|   IBIS model for TI xxx DSP
[IBIS Ver]   5.1
[Disclaimer]   Please be aware that in the absence of a written agreement
|   Texas Instruments(TI) assumes no liability for:
|   (1) The accuracy of the IBIS models provided to your company,
|   however, the IBIS model is compliant to industry standard
|   IQ Level 2a.  Refer to IBIS Quality Section below for
|   for full details.
|   (2) The proper functioning of these Models in your design
|   or for any resulting applications
|   (3) Infringement of patents, copyrights or intellectual
|   property rights resulting from your use of these
|   models.
|   TI provides IBIS Models as a service to our customers and
|   therefore reserves the right to limit distribution of the
|   Models.  The information is subject to change without notice.
[File Name]  j7es_v0p2.ibs
[File Rev]   0.2
|   - 0.1: Initial version
|   - 0.2: Added Package Model section in J7ES component
[Date]   28 August 2019
[Source]   Texas Instruments Incorporated
[Copyright]   Property of Texas Instruments Incorporated.
|   Unauthorized reproduction and/or distribution is strictly.
|   prohibited.
|   This product is protected under copyright law and trade
|   secret law as an unpublished work.
|   Created 2012,(C) Copyright 1999-2012,
|   Texas Instruments Incorporated., All Rights Reserved.
|   These commodities are under the U.S. Government
|   distribution license control. As such,they are not to be
|   re-exported without the prior approval of the U.S.
|   Department of Commerce.
[Notes]
   This file does not include AMI models for the following:
   1. PCIe
   2. CSI
   3. Display Port
   4. USB2
   5. USB3
   6. MPHY
   For SerDes simulations use Texas Instruments IBIS AMI models
   Some IV curves contain Non monotonic data points.
|   Revision History
|   GERNERAL COMMENT: All IBIS Quality Notes below reflect latest release
|   and version of IBIS File
|   File passes ibischk6.0 with 0 errors and 112 warnings
|   Component J7ES
[Component] J7ES
[Manufacturer] Texas Instruments
[Package Model] ibis_j7es_sck_181218
[Package]
|Variable   Typ   Min   Max
R_pkg   0.16518   0.088878   0.23503
L_pkg   1.464e-9   1.019e-9   2.221e-9
C_pkg   1.572e-12   1.113e-12   1.967e-12
[Pin]  Signal_name   model_name
AJ29	ATEST0   NC
U7	CAP_VDDS0   POWER
K23	CAP_VDDS0_MCU   POWER
AB21	CAP_VDDS1   POWER
J18	CAP_VDDS1_MCU   POWER
Y18	CAP_VDDS2   POWER
J19	CAP_VDDS2_MCU   POWER
W21	CAP_VDDS3   POWER
AA22	CAP_VDDS4   POWER
R22	CAP_VDDS5   POWER
V22	CAP_VDDS6   POWER
T11	CC12   NC
T12	CC12   NC
T13	CC12   NC
U11	CC12   NC
U12	CC12   NC
U13	CC12   NC
M11	CC34   NC
M12	CC34   NC
M13	CC34   NC
N11	CC34   NC
N12	CC34   NC
N13	CC34   NC
E18	CSI0_ATB_0_H   NC
F18	CSI0_ATB_1_H   NC
B20	CSI0_RXCLKN   NC
A21	CSI0_RXCLKP   NC
B19	CSI0_RXN0   NC
D18	CSI0_RXN1   NC
D17	CSI0_RXN2   NC
E16	CSI0_RXN3   NC
A20	CSI0_RXP0   NC
C19	CSI0_RXP1   NC
C18	CSI0_RXP2   NC
E17	CSI0_RXP3   NC
F16	csi0_rxrcalib   NC
G10	csi1_atb_0_h   NC
F11	csi1_atb_1_h   NC
B17	CSI1_RXCLKN   NC
A18	CSI1_RXCLKP   NC
B16	CSI1_RXN0   NC
D15	CSI1_RXN1   NC
D14	CSI1_RXN2   NC
E13	CSI1_RXN3   NC
A17	CSI1_RXP0   NC
C16	CSI1_RXP1   NC
C15	CSI1_RXP2   NC
E14	CSI1_RXP3   NC
F15	csi1_rxrcalib   NC
P6	ddr_ret   NC
N6	ddr0_atb0   NC
L6	ddr0_atb1   NC
G4	ddr0_ca0	DDR_SE
H3	ddr0_ca1	DDR_SE
K5	ddr0_ca2	DDR_SE
J4	ddr0_ca3	DDR_SE
K2	ddr0_ca4	DDR_SE
H5	ddr0_ca5	DDR_SE
H2	ddr0_cal0	DDR_SE
G3	ddr0_cke0	DDR_SE
J3	ddr0_cke1	DDR_SE
J1	ddr0_ckn	DDR_DIFF
H1	ddr0_ckp	DDR_DIFF
J5	ddr0_csn0_0	DDR_SE
K3	ddr0_csn0_1	DDR_SE
G5	ddr0_csn1_0	DDR_SE
J2	ddr0_csn1_1	DDR_SE
A3	ddr0_dm0	DDR_SE
E4	ddr0_dm1	DDR_SE
N1	ddr0_dm2	DDR_SE
R5	ddr0_dm3	DDR_SE
A5	ddr0_dq0	DDR_SE
A6	ddr0_dq1	DDR_SE
F1	ddr0_dq10	DDR_SE
G2	ddr0_dq11	DDR_SE
F2	ddr0_dq12	DDR_SE
F3	ddr0_dq13	DDR_SE
D3	ddr0_dq14	DDR_SE
F5	ddr0_dq15	DDR_SE
L5	ddr0_dq16	DDR_SE
M5	ddr0_dq17	DDR_SE
N5	ddr0_dq18	DDR_SE
L4	ddr0_dq19	DDR_SE
B5	ddr0_dq2	DDR_SE
L2	ddr0_dq20	DDR_SE
L1	ddr0_dq21	DDR_SE
N2	ddr0_dq22	DDR_SE
N4	ddr0_dq23	DDR_SE
T3	ddr0_dq24	DDR_SE
T2	ddr0_dq25	DDR_SE
P2	ddr0_dq26	DDR_SE
P3	ddr0_dq27	DDR_SE
P5	ddr0_dq28	DDR_SE
R4	ddr0_dq29	DDR_SE
C2	ddr0_dq3	DDR_SE
T4	ddr0_dq30	DDR_SE
T5	ddr0_dq31	DDR_SE
B4	ddr0_dq4	DDR_SE
C3	ddr0_dq5	DDR_SE
A2	ddr0_dq6	DDR_SE
A4	ddr0_dq7	DDR_SE
D1	ddr0_dq8	DDR_SE
C4	ddr0_dq9	DDR_SE
B1	ddr0_dqs0n	DDR_DIFF
B2	ddr0_dqs0p	DDR_DIFF
E2	ddr0_dqs1n	DDR_DIFF
E3	ddr0_dqs1p	DDR_DIFF
M2	ddr0_dqs2n	DDR_DIFF
M3	ddr0_dqs2p	DDR_DIFF
R1	ddr0_dqs3n	DDR_DIFF
R2	ddr0_dqs3p	DDR_DIFF
K6	ddr0_resetn	DDR_SE
F6	dp0_aux_atb_0   NC
E6	dp0_aux_atb_1   NC
G6	dp0_auxn   NC
F7	dp0_auxp   NC
G9	dsi_atb_0_h   NC
F10	dsi_atb_1_h   NC
E10	DSI_TXCLKN	NC
E11	DSI_TXCLKP	NC
D11	DSI_TXN0	NC
D12	DSI_TXN1	NC
B13	DSI_TXN2	NC
B14	DSI_TXN3	NC
C12	DSI_TXP0	NC
C13	DSI_TXP1	NC
A14	DSI_TXP2	NC
A15	DSI_TXP3	NC
F12	dsi_txrcalib	NC
U2	ecap0_in_apwm_out	LVCMOS_H
C26	emu0	LVCMOS_H
B29	emu1	LVCMOS_H
U3	ext_refclk1	LVCMOS_H
AC18	extintn	LVCMOS_V
AC5	i2c0_scl	IIC_H
AA5	i2c0_sda	IIC_H
Y6	i2c1_scl	IIC_H
AA6	i2c1_sda	IIC_H
W2	i3c0_scl	LVCMOS_H
W1	i3c0_sda	LVCMOS_H
P26	iforce	NC
N25	MAIN_ATEST	NC
W5	mcan0_rx	LVCMOS_H
W6	mcan0_tx	LVCMOS_H
W3	mcan1_rx	LVCMOS_H
V4	mcan1_tx	LVCMOS_H
K25	mcu_adc0_ain0	NC
K26	mcu_adc0_ain1	NC
K28	mcu_adc0_ain2	NC
L28	mcu_adc0_ain3	NC
K24	mcu_adc0_ain4	NC
K27	mcu_adc0_ain5	NC
K29	mcu_adc0_ain6	NC
L29	mcu_adc0_ain7	NC
N23	mcu_adc1_ain0	NC
M25	mcu_adc1_ain1	NC
L24	mcu_adc1_ain2	NC
L26	mcu_adc1_ain3	NC
N24	mcu_adc1_ain4	NC
M24	mcu_adc1_ain5	NC
L25	mcu_adc1_ain6	NC
L27	mcu_adc1_ain7	NC
J26	mcu_i2c0_scl	IIC_H
H25	mcu_i2c0_sda	IIC_H
D26	mcu_i3c0_scl	LVCMOS_H
D25	mcu_i3c0_sda	LVCMOS_H
C29	mcu_mcan0_rx	LVCMOS_H
D29	mcu_mcan0_tx	LVCMOS_H
F23	mcu_mdio0_mdc	LVCMOS_H
E23	mcu_mdio0_mdio	LVCMOS_H
E20	mcu_ospi0_clk	LVCMOS_V
F19	mcu_ospi0_csn0	LVCMOS_V
E19	mcu_ospi0_csn1	LVCMOS_V
D20	mcu_ospi0_d0	LVCMOS_V
G19	mcu_ospi0_d1	LVCMOS_V
G20	mcu_ospi0_d2	LVCMOS_V
F20	mcu_ospi0_d3	LVCMOS_V
F21	mcu_ospi0_d4	LVCMOS_V
E21	mcu_ospi0_d5	LVCMOS_V
B22	mcu_ospi0_d6	LVCMOS_V
G21	mcu_ospi0_d7	LVCMOS_V
D21	mcu_ospi0_dqs	LVCMOS_V
C21	mcu_ospi0_lbclko	LVCMOS_V
F22	mcu_ospi1_clk	LVCMOS_V
C22	mcu_ospi1_csn0	LVCMOS_V
E22	mcu_ospi1_csn1	LVCMOS_V
D22	mcu_ospi1_d0	LVCMOS_V
G22	mcu_ospi1_d1	LVCMOS_V
D23	mcu_ospi1_d2	LVCMOS_V
C23	mcu_ospi1_d3	LVCMOS_V
B23	mcu_ospi1_dqs	LVCMOS_V
A23	mcu_ospi1_lbclko	LVCMOS_V
H23	mcu_porz	RESET_H
B28	mcu_porz_out	LVCMOS_H
C27	mcu_resetstatz	LVCMOS_H
D28	mcu_resetz	LVCMOS_H
B24	mcu_rgmii1_rd0	LVCMOS_H
A24	mcu_rgmii1_rd1	LVCMOS_H
D24	mcu_rgmii1_rd2	LVCMOS_H
A25	mcu_rgmii1_rd3	LVCMOS_H
C25	mcu_rgmii1_rx_ctl	LVCMOS_H
C24	mcu_rgmii1_rxc	LVCMOS_H
B25	mcu_rgmii1_td0	LVCMOS_H
A26	mcu_rgmii1_td1	LVCMOS_H
A27	mcu_rgmii1_td2	LVCMOS_H
A28	mcu_rgmii1_td3	LVCMOS_H
B27	mcu_rgmii1_tx_ctl	LVCMOS_H
B26	mcu_rgmii1_txc	LVCMOS_H
D27	mcu_safety_errorn	LVCMOS_H
E27	mcu_spi0_clk	LVCMOS_H
E25	mcu_spi0_cs0	LVCMOS_H
E24	mcu_spi0_d0	LVCMOS_H
E28	mcu_spi0_d1	LVCMOS_H
V24	mdio0_mdc	LVCMOS_H
V26	mdio0_mdio	LVCMOS_H
AE2	mlb0_mlbcn	LVDS
AD2	mlb0_mlbcp	LVDS
AD3	mlb0_mlbdn	LVDS
AC3	mlb0_mlbdp	LVDS
AC1	mlb0_mlbsn	LVDS
AD1	mlb0_mlbsp	LVDS
AE1	mmc0_calpad	EMMC
AF1	mmc0_clk	EMMC
AE3	mmc0_cmd	EMMC
AG2	mmc0_dat0	EMMC
AH1	mmc0_dat1	EMMC
AG3	mmc0_dat2	EMMC
AF4	mmc0_dat3	EMMC
AE5	mmc0_dat4	EMMC
AF3	mmc0_dat5	EMMC
AG1	mmc0_dat6	EMMC
AF2	mmc0_dat7	EMMC
AE4	mmc0_ds   EMMC
AD4	mmc0_vctrl_tp	EMMC
P25	mmc1_clk	SDIO_H
R29	mmc1_cmd	SDIO_H
R24	mmc1_dat0	SDIO_H
P24	mmc1_dat1	SDIO_H
R25	mmc1_dat2	SDIO_H
R26	mmc1_dat3	SDIO_H
P23	mmc1_sdcd	LVCMOS_H
R28	mmc1_sdwp	LVCMOS_H
T26	mmc2_clk	SDIO_H
T25	mmc2_cmd	SDIO_H
T24	mmc2_dat0	SDIO_H
T27	mmc2_dat1	SDIO_H
T29	mmc2_dat2	SDIO_H
T28	mmc2_dat3	SDIO_H
P29	osc1_xi	NC
P27	osc1_xo	NC
AE17	pcie_refclk0n	NC
AD16	pcie_refclk0p	NC
AE14	pcie_refclk1n	NC
AD15	pcie_refclk1p	NC
AE11	pcie_refclk2n	NC
AD12	pcie_refclk2p	NC
AE9	pcie_refclk3n	NC
AD10	pcie_refclk3p	NC
E26	pmic_power_en0	LVCMOS_H
G23	pmic_power_en1	LVCMOS_H
J24	porz   RESET_H
U1	porz_out	LVCMOS_H
AA27	prg0_mdio0_mdc	LVCMOS_V
Y26	prg0_mdio0_mdio	LVCMOS_V
AF28	prg0_pru0_gpo0	LVCMOS_V
AE28	prg0_pru0_gpo1	LVCMOS_V
AB25	prg0_pru0_gpo10	LVCMOS_V
AJ28	prg0_pru0_gpo11	LVCMOS_V
AH27	prg0_pru0_gpo12	LVCMOS_V
AH29	prg0_pru0_gpo13	LVCMOS_V
AG28	prg0_pru0_gpo14	LVCMOS_V
AG27	prg0_pru0_gpo15	LVCMOS_V
AH28	prg0_pru0_gpo16	LVCMOS_V
AB24	prg0_pru0_gpo17	LVCMOS_V
AB29	prg0_pru0_gpo18	LVCMOS_V
AB28	prg0_pru0_gpo19	LVCMOS_V
AE27	prg0_pru0_gpo2	LVCMOS_V
AD26	prg0_pru0_gpo3	LVCMOS_V
AD25	prg0_pru0_gpo4	LVCMOS_V
AC29	prg0_pru0_gpo5	LVCMOS_V
AE26	prg0_pru0_gpo6	LVCMOS_V
AC28	prg0_pru0_gpo7	LVCMOS_V
AC27	prg0_pru0_gpo8	LVCMOS_V
AB26	prg0_pru0_gpo9	LVCMOS_V
AE29	prg0_pru1_gpo0	LVCMOS_V
AD28	prg0_pru1_gpo1	LVCMOS_V
AA25	prg0_pru1_gpo10	LVCMOS_V
AG26	prg0_pru1_gpo11	LVCMOS_V
AF27	prg0_pru1_gpo12	LVCMOS_V
AF26	prg0_pru1_gpo13	LVCMOS_V
AE25	prg0_pru1_gpo14	LVCMOS_V
AF29	prg0_pru1_gpo15	LVCMOS_V
AG29	prg0_pru1_gpo16	LVCMOS_V
Y25	prg0_pru1_gpo17	LVCMOS_V
AA26	prg0_pru1_gpo18	LVCMOS_V
AA29	prg0_pru1_gpo19	LVCMOS_V
AD27	prg0_pru1_gpo2	LVCMOS_V
AC25	prg0_pru1_gpo3	LVCMOS_V
AD29	prg0_pru1_gpo4	LVCMOS_V
AB27	prg0_pru1_gpo5	LVCMOS_V
AC26	prg0_pru1_gpo6	LVCMOS_V
AA24	prg0_pru1_gpo7	LVCMOS_V
AA28	prg0_pru1_gpo8	LVCMOS_V
Y24	prg0_pru1_gpo9	LVCMOS_V
AD18	prg1_mdio0_mdc	LVCMOS_V
AD19	prg1_mdio0_mdio	LVCMOS_V
AC23	prg1_pru0_gpo0	LVCMOS_V
AG22	prg1_pru0_gpo1	LVCMOS_V
AD21	prg1_pru0_gpo10	LVCMOS_V
AF24	prg1_pru0_gpo11	LVCMOS_V
AJ24	prg1_pru0_gpo12	LVCMOS_V
AG24	prg1_pru0_gpo13	LVCMOS_V
AD24	prg1_pru0_gpo14	LVCMOS_V
AC24	prg1_pru0_gpo15	LVCMOS_V
AE24	prg1_pru0_gpo16	LVCMOS_V
AJ21	prg1_pru0_gpo17	LVCMOS_V
AE21	prg1_pru0_gpo18	LVCMOS_V
AH21	prg1_pru0_gpo19	LVCMOS_V
AF22	prg1_pru0_gpo2	LVCMOS_V
AJ23	prg1_pru0_gpo3	LVCMOS_V
AH23	prg1_pru0_gpo4	LVCMOS_V
AD20	prg1_pru0_gpo5	LVCMOS_V
AD22	prg1_pru0_gpo6	LVCMOS_V
AE20	prg1_pru0_gpo7	LVCMOS_V
AJ20	prg1_pru0_gpo8	LVCMOS_V
AG20	prg1_pru0_gpo9	LVCMOS_V
AE22	prg1_pru1_gpo0	LVCMOS_V
AG23	prg1_pru1_gpo1	LVCMOS_V
AB23	prg1_pru1_gpo10	LVCMOS_V
AJ25	prg1_pru1_gpo11	LVCMOS_V
AH25	prg1_pru1_gpo12	LVCMOS_V
AG25	prg1_pru1_gpo13	LVCMOS_V
AH26	prg1_pru1_gpo14	LVCMOS_V
AJ27	prg1_pru1_gpo15	LVCMOS_V
AJ26	prg1_pru1_gpo16	LVCMOS_V
AC22	prg1_pru1_gpo17	LVCMOS_V
AJ22	prg1_pru1_gpo18	LVCMOS_V
AH22	prg1_pru1_gpo19	LVCMOS_V
AF23	prg1_pru1_gpo2	LVCMOS_V
AD23	prg1_pru1_gpo3	LVCMOS_V
AH24	prg1_pru1_gpo4	LVCMOS_V
AG21	prg1_pru1_gpo5	LVCMOS_V
AE23	prg1_pru1_gpo6	LVCMOS_V
AC21	prg1_pru1_gpo7	LVCMOS_V
Y23	prg1_pru1_gpo8	LVCMOS_V
AF21	prg1_pru1_gpo9	LVCMOS_V
C28	RESET_REQZ	LVCMOS_H
T6	resetstatz	LVCMOS_H
T23	rgmii5_rd0	LVCMOS_H
R23	rgmii5_rd1	LVCMOS_H
U24	rgmii5_rd2	LVCMOS_H
U27	rgmii5_rd3	LVCMOS_H
U26	rgmii5_rx_ctl	LVCMOS_H
U25	rgmii5_rxc	LVCMOS_H
U28	rgmii5_td0	LVCMOS_H
V27	rgmii5_td1	LVCMOS_H
V29	rgmii5_td2	LVCMOS_H
V28	rgmii5_td3	LVCMOS_H
U23	rgmii5_tx_ctl	LVCMOS_H
U29	rgmii5_txc	LVCMOS_H
W25	rgmii6_rd0	LVCMOS_H
W24	rgmii6_rd1	LVCMOS_H
Y27	rgmii6_rd2	LVCMOS_H
Y29	rgmii6_rd3	LVCMOS_H
V23	rgmii6_rx_ctl	LVCMOS_H
W26	rgmii6_rxc	LVCMOS_H
W27	rgmii6_td0	LVCMOS_H
V25	rgmii6_td1	LVCMOS_H
W28	rgmii6_td2	LVCMOS_H
W23	rgmii6_td3	LVCMOS_H
Y28	rgmii6_tx_ctl	LVCMOS_H
W29	rgmii6_txc	LVCMOS_H
AE18	serdes0_rext	NC
AH19	SERDES0_RX0_N	NC
AJ18	SERDES0_RX0_P	NC
AH18	SERDES0_RX1_N	NC
AJ17	SERDES0_RX1_P	NC
AF19	SERDES0_TX0_N	NC
AG18	SERDES0_TX0_P	NC
AF18	SERDES0_TX1_N	NC
AG17	SERDES0_TX1_P	NC
AE13	serdes1_rext	NC
AH15	SERDES1_RX0_N	NC
AJ14	SERDES1_RX0_P	NC
AH16	SERDES1_RX1_N	NC
AJ15	SERDES1_RX1_P	NC
AF15	SERDES1_TX0_N	NC
AG14	SERDES1_TX0_P	NC
AF16	SERDES1_TX1_N	NC
AG15	SERDES1_TX1_P	NC
AD13	serdes2_rext	NC
AH13	SERDES2_RX0_N	NC
AJ12	SERDES2_RX0_P	NC
AH12	SERDES2_RX1_N	NC
AJ11	SERDES2_RX1_P	NC
AF13	SERDES2_TX0_N	NC
AG12	SERDES2_TX0_P	NC
AF12	SERDES2_TX1_N	NC
AG11	SERDES2_TX1_P	NC
AE8	serdes3_rext	NC
AH9	SERDES3_RX0_N	NC
AJ8	SERDES3_RX0_P	NC
AH10	SERDES3_RX1_N	NC
AJ9	SERDES3_RX1_P	NC
AF9	SERDES3_TX0_N	NC
AG8	SERDES3_TX0_P	NC
AF10	SERDES3_TX1_N	NC
AG9	SERDES3_TX1_P	NC
E7	SERDES4_REFCLK_N	NC
E8	SERDES4_REFCLK_P	NC
F9	serdes4_rext	NC
D9	SERDES4_RX0_N	NC
C10	SERDES4_RX0_P	NC
D8	SERDES4_RX1_N	NC
C9	SERDES4_RX1_P	NC
D6	SERDES4_RX2_N	NC
C7	SERDES4_RX2_P	NC
D5	SERDES4_RX3_N	NC
C6	SERDES4_RX3_P	NC
B11	SERDES4_TX0_N	NC
A12	SERDES4_TX0_P	NC
B10	SERDES4_TX1_N	NC
A11	SERDES4_TX1_P	NC
B8	SERDES4_TX2_N	NC
A9	SERDES4_TX2_P	NC
B7	SERDES4_TX3_N	NC
A8	SERDES4_TX3_P	NC
U4	soc_safety_errorn	LVCMOS_H
AA1	spi0_clk   LVCMOS_H
AA2	spi0_cs0   LVCMOS_H
Y4	spi0_cs1   LVCMOS_H
AB5	spi0_d0   LVCMOS_H
AA3	spi0_d1   LVCMOS_H
Y1	spi1_clk   LVCMOS_H
Y3	spi1_cs0   LVCMOS_H
W4	spi1_cs1   LVCMOS_H
Y5	spi1_d0   LVCMOS_H
Y2	spi1_d1   LVCMOS_H
E29	tck   LVCMOS_H
V1	tdi   LVCMOS_H
V3	tdo   LVCMOS_H
F13	temp_diode_p   NC
V6	timer_io0   LVCMOS_H
V5	timer_io1   LVCMOS_H
V2	tms   LVCMOS_H
F24	trstn   LVCMOS_H
AC2	uart0_ctsn	LVCMOS_H
AB1	uart0_rtsn	LVCMOS_H
AB2	uart0_rxd	LVCMOS_H
AB3	uart0_txd	LVCMOS_H
AC4	uart1_ctsn	LVCMOS_H
AD5	uart1_rtsn	LVCMOS_H
AA4	uart1_rxd	LVCMOS_H
AB4	uart1_txd	LVCMOS_H
AE6	ufs0_ref_clk	NC
AD6	ufs0_rstn	NC
AH3	ufs0_rx_dn0	NC
AH4	ufs0_rx_dn1	NC
AJ2	ufs0_rx_dp0	NC
AJ3	ufs0_rx_dp1	NC
AG6	ufs0_tx_dn0	NC
AG5	ufs0_tx_dn1	NC
AF7	ufs0_tx_dp0	NC
AF6	ufs0_tx_dp1	NC
AJ5	usb0_dm   NC
AH6	usb0_dp   NC
U6	usb0_drvvbus	LVCMOS_H
AC6	usb0_id   NC
AB6	usb0_rcalib	NC
AC7	usb0_vbus   NC
AH7	usb1_dm   NC
AJ6	usb1_dp   NC
AD7	usb1_id   NC
AD9	usb1_rcalib   NC
AD8	usb1_vbus	NC
J10	VDD_CORE	POWER
K9	VDD_CORE	POWER
K11	VDD_CORE	POWER
K13	VDD_CORE	POWER
K15	VDD_CORE	POWER
K17	VDD_CORE	POWER
L10	VDD_CORE	POWER
L16	VDD_CORE	POWER
L18	VDD_CORE	POWER
M15	VDD_CORE	POWER
N14	VDD_CORE	POWER
N16	VDD_CORE	POWER
N18	VDD_CORE	POWER
P13	VDD_CORE	POWER
P15	VDD_CORE	POWER
P17	VDD_CORE	POWER
R14	VDD_CORE	POWER
R16	VDD_CORE	POWER
R18	VDD_CORE	POWER
R20	VDD_CORE	POWER
T9	VDD_CORE	POWER
T15	VDD_CORE	POWER
T17	VDD_CORE	POWER
U14	VDD_CORE	POWER
U16	VDD_CORE	POWER
U18	VDD_CORE	POWER
V15	VDD_CORE	POWER
V17	VDD_CORE	POWER
V20	VDD_CORE	POWER
W14	VDD_CORE	POWER
N10	VDD_CPU   POWER
P11	VDD_CPU   POWER
R10	VDD_CPU   POWER
R12	VDD_CPU   POWER
U10	VDD_CPU   POWER
V9	VDD_CPU   POWER
V11	VDD_CPU   POWER
W10	VDD_CPU   POWER
Y9	VDD_DLL_MMC0	POWER
L20	vdd_mcu   POWER
M19	vdd_mcu   POWER
M21	vdd_mcu   POWER
N20	vdd_mcu   POWER
P19	vdd_mcu   POWER
V19	VDD_VMON_EXT_MON	POWER
H17	VDDA_0P8_CSIRX	POWER
G12	VDDA_0P8_DP	POWER
J12	VDDA_0P8_DP	POWER
G14	VDDA_0P8_DP_C	POWER
H13	VDDA_0P8_DP_C	POWER
H15	VDDA_0P8_DSITX	POWER
J16	VDDA_0P8_DSITX_C	POWER
AB14	VDDA_0P8_SERDES_C0_1	POWER
AB15	VDDA_0P8_SERDES_C0_1	POWER
AB12	VDDA_0P8_SERDES_C2_3	POWER
AB13	VDDA_0P8_SERDES_C2_3	POWER
Y14	VDDA_0P8_SERDES0_1	POWER
Y16	VDDA_0P8_SERDES0_1	POWER
AA15	VDDA_0P8_SERDES0_1	POWER
Y11	VDDA_0P8_SERDES2_3	POWER
Y13	VDDA_0P8_SERDES2_3	POWER
AA12	VDDA_0P8_SERDES2_3	POWER
AB9	VDDA_0P8_UFS	POWER
AA10	VDDA_0P8_USB	POWER
G16	VDDA_1P8_CSIRX	POWER
H11	VDDA_1P8_DP	POWER
J14	VDDA_1P8_DSITX	POWER
AC14	VDDA_1P8_SERDES0_1	POWER
AC15	VDDA_1P8_SERDES0_1	POWER
AC11	VDDA_1P8_SERDES2_3	POWER
AC12	VDDA_1P8_SERDES2_3	POWER
AC8	VDDA_1P8_UFS	POWER
AC9	vdda_1p8_usb	POWER
AB10	vdda_3p3_usb	POWER
N22	VDDA_ADC0	POWER
M23	VDDA_ADC1	POWER
N9	VDDA_DDR_PLL	POWER
G18	VDDA_MCU_PLLGRP0	POWER
P21	VDDA_MCU_TEMP	POWER
W7	VDDA_MLB	POWER
Y20	VDDA_PLLGRP0	POWER
W17	VDDA_PLLGRP1	POWER
M17	VDDA_PLLGRP2	POWER
L12	VDDA_PLLGRP3	POWER
R11	VDDA_PLLGRP4	POWER
P9	VDDA_PLLGRP5	POWER
W18	VDDA_PLLGRP6	POWER
W8	VDDA_PLLGRP7	POWER
P22	vdda_por_wkup	POWER
W15	VDDA_TEMP0_1	POWER
H9	VDDA_TEMP2_3	POWER
M26	VDDA_VSYS_MON	POWER
H22	VDDA_WKUP	POWER
L14	VDDAR_CORE	POWER
V13	VDDAR_CORE	POWER
V16	VDDAR_CORE	POWER
W19	VDDAR_CORE	POWER
L11	VDDAR_CPU	POWER
W12	VDDAR_CPU	POWER
K19	vddar_mcu	POWER
T19	vddar_mcu	POWER
A1	vdds_ddr	POWER
G8	vdds_ddr	POWER
J8	vdds_ddr	POWER
K7	vdds_ddr	POWER
L8	vdds_ddr	POWER
M7	vdds_ddr	POWER
N8	vdds_ddr	POWER
P7	vdds_ddr	POWER
R8	vdds_ddr	POWER
T1	vdds_ddr	POWER
H7	vdds_ddr_bias	POWER
J6	vdds_ddr_bias	POWER
R6	vdds_ddr_bias	POWER
T7	vdds_ddr_bias	POWER
M9	VDDS_DDR_C	POWER
Y7	vdds_mmc0	POWER
AA8	vdds_mmc0	POWER
AB7	vdds_mmc0	POWER
R21	VDDS_OSC1	POWER
U8	VDDSHV0   POWER
V7	VDDSHV0   POWER
L22	VDDSHV0_MCU	POWER
M22	VDDSHV0_MCU	POWER
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|********************  DIFF PIN  *******************************
[Diff_pin]   inv_pin vdiff tdelay_typ   tdelay_min  tdelay_max
B1	B2	NA NA NA NA	||	ddr0_dqs0n	&	ddr0_dqs0p
E2	E3	NA NA NA NA	||	ddr0_dqs1n	&	ddr0_dqs1p
M2	M3	NA NA NA NA	||	ddr0_dqs2n	&	ddr0_dqs2p
R1	R2	NA NA NA NA	||	ddr0_dqs3n	&	ddr0_dqs3p
J1	H1	NA NA NA NA	||	ddr0_ckn	&	ddr0_ckp
[Series Pin Mapping] pin_2 model_name function_table_group
| AC25	AD25	s_ILVDS18TH_PB300
| AD24	AE24	s_ILVDS18TH_PB300
| K21	L21	s_ILVDS18TH_PB300
|---------------- DDR -------------------
[Model Selector] DDR_SE
lpddr4_ocd_240p_240n  driver with 240 ohms pullup and 240 ohms pulldown strength
lpddr4_ocd_120p_120n  driver with 120 ohms pullup and 120 ohms pulldown strength
lpddr4_ocd_80p_80n  driver with 80 ohms pullup and 80 ohms pulldown strength
lpddr4_ocd_60p_60n  driver with 60 ohms pullup and 60 ohms pulldown strength
lpddr4_ocd_48p_48n  driver with 48 ohms pullup and 48 ohms pulldown strength
lpddr4_ocd_40p_40n  driver with 40 ohms pullup and 40 ohms pulldown strength
lpddr4_ocd_120pd_60p_40n  driver with 60/40 ohms pullup/pulldown 120 ohms aopd strength
lpddr4_ocd_120pd_48p_40n  driver with 48/40 ohms pullup/pulldown 120 ohms aopd strength
lp4x_ocd_34p_34n  driver with 34 ohms pullup and 34 ohms pulldown strength
lp4x_ocd_40p_40n  driver with 40 ohms pullup and 40 ohms pulldown strength
lp4x_ocd_48p_48n  driver with 48 ohms pullup and 48 ohms pulldown strength
lp4x_ocd_60p_60n  driver with 60 ohms pullup and 60 ohms pulldown strength
lp4x_ocd_80p_80n  driver with 80 ohms pullup and 80 ohms pulldown strength
lp4x_ocd_120p_120n  driver with 120 ohms pullup and 120 ohms pulldown strength
lp4x_ocd_240p_240n  driver with 240 ohms pullup and 240 ohms pulldown strength
lp4x_0p6_ocd_80p_80n  driver with 80 ohms pullup and 80 ohms pulldown strength
lp4x_0p6_ocd_40p_40n  driver with 40 ohms pullup and 40 ohms pulldown strength
lpddr4_odt_240  240 ohm termination
lpddr4_odt_120  120 ohm termination
lpddr4_odt_80  80 ohm termination
lpddr4_odt_60  60 ohm termination
lpddr4_odt_48  48 ohm termination
lpddr4_odt_40  40 ohm termination
lpddr4_odt_off  open ohm termination
lp4x_odt_40  40 ohm termination
lp4x_odt_48  48 ohm termination
lp4x_odt_60  60 ohm termination
lp4x_odt_80  80 ohm termination
lp4x_odt_120  120 ohm termination
lp4x_odt_240  240 ohm termination
lp4x_odt_off  open
[Model Selector] DDR_DIFF
lpddr4_ocd_240p_240n_diff  driver with 240 ohms pullup and 240 ohms pulldown strength
lpddr4_ocd_120p_120n_diff  driver with 120 ohms pullup and 120 ohms pulldown strength
lpddr4_ocd_80p_80n_diff  driver with 80 ohms pullup and 80 ohms pulldown strength
lpddr4_ocd_60p_60n_diff  driver with 60 ohms pullup and 60 ohms pulldown strength
lpddr4_ocd_48p_48n_diff  driver with 48 ohms pullup and 48 ohms pulldown strength
lpddr4_ocd_40p_40n_diff  driver with 40 ohms pullup and 40 ohms pulldown strength
lpddr4_ocd_120pd_60p_40n_diff  driver with 60/40 ohms pullup/pulldown 120 ohms aopd strength
lpddr4_ocd_120pd_48p_40n_diff  driver with 48/40 ohms pullup/pulldown 120 ohms aopd strength
lp4x_ocd_34p_34n_diff  driver with 34 ohms pullup and 34 ohms pulldown strength
lp4x_ocd_40p_40n_diff  driver with 40 ohms pullup and 40 ohms pulldown strength
lp4x_ocd_48p_48n_diff  driver with 48 ohms pullup and 48 ohms pulldown strength
lp4x_ocd_60p_60n_diff  driver with 60 ohms pullup and 60 ohms pulldown strength
lp4x_ocd_80p_80n_diff  driver with 80 ohms pullup and 80 ohms pulldown strength
lp4x_ocd_120p_120n_diff  driver with 120 ohms pullup and 120 ohms pulldown strength
lp4x_ocd_240p_240n_diff  driver with 240 ohms pullup and 240 ohms pulldown strength
lp4x_0p6_ocd_80p_80n_diff  driver with 80 ohms pullup and 80 ohms pulldown strength
lp4x_0p6_ocd_40p_40n_diff  driver with 40 ohms pullup and 40 ohms pulldown strength
lpddr4_odt_240_diff  240 ohm termination
lpddr4_odt_120_diff  120 ohm termination
lpddr4_odt_80_diff  80 ohm termination
lpddr4_odt_60_diff  60 ohm termination
lpddr4_odt_48_diff  48 ohm termination
lpddr4_odt_40_diff  40 ohm termination
lpddr4_odt_off_diff  open ohm termination
lp4x_odt_40_diff  40 ohm termination
lp4x_odt_48_diff  48 ohm termination
lp4x_odt_60_diff  60 ohm termination
lp4x_odt_80_diff  80 ohm termination
lp4x_odt_120_diff  120 ohm termination
lp4x_odt_240_diff  240 ohm termination
lp4x_odt_off_diff  open
|****************** SDIO
[Model Selector] SDIO_H
sdio1_r33_1p8_h PRWDWUWSWEWCDGSDIO_H@_R33_1p8_comment
sdio1_r33_3p3_h PRWDWUWSWEWCDGSDIO_H@_R33_3p3_comment
sdio1_r40_1p8_h PRWDWUWSWEWCDGSDIO_H@_R40_1p8_comment
sdio1_r40_3p3_h PRWDWUWSWEWCDGSDIO_H@_R40_3p3_comment
sdio1_r50_1p8_h PRWDWUWSWEWCDGSDIO_H@_R50_1p8_comment
sdio1_r50_3p3_h PRWDWUWSWEWCDGSDIO_H@_R50_3p3_comment
sdio1_r66_1p8_h PRWDWUWSWEWCDGSDIO_H@_R66_1p8_comment
sdio1_r66_3p3_h PRWDWUWSWEWCDGSDIO_H@_R66_3p3_comment
sdio1_utr33_1p8_h PRWDWUWSWEWCDGSDIO_H@_UT_R33_1p8_comment
sdio1_utr33_3p3_h PRWDWUWSWEWCDGSDIO_H@_UT_R33_3p3_comment
sdio1_utr40_1p8_h PRWDWUWSWEWCDGSDIO_H@_UT_R40_1p8_comment
sdio1_utr40_3p3_h PRWDWUWSWEWCDGSDIO_H@_UT_R40_3p3_comment
sdio1_utr50_1p8_h PRWDWUWSWEWCDGSDIO_H@_UT_R50_1p8_comment
sdio1_utr50_3p3_h PRWDWUWSWEWCDGSDIO_H@_UT_R50_3p3_comment
sdio1_utr66_1p8_h PRWDWUWSWEWCDGSDIO_H@_UT_R66_1p8_comment
sdio1_utr66_3p3_h PRWDWUWSWEWCDGSDIO_H@_UT_R66_3p3_comment
|********** LVCMOS
[Model Selector] LVCMOS_H
lvcmos1_nom_1p8_h PRWDWUWSWEWCDGLVCMOS_H@_Nom_1p8_comment
lvcmos1_nom_3p3_h PRWDWUWSWEWCDGLVCMOS_H@_Nom_3p3_comment
lvcmos1_slow_1p8_h PRWDWUWSWEWCDGLVCMOS_H@_Slow_1p8_comment
lvcmos1_slow_3p3_h PRWDWUWSWEWCDGLVCMOS_H@_Slow_3p3_comment
lvcmos1_fast_1p8_h PRWDWUWSWEWCDGLVCMOS_H@_Fast_1p8_comment
lvcmos1_fast_3p3_h PRWDWUWSWEWCDGLVCMOS_H@_Fast_3p3_comment
lvcmos1_utnom_1p8_h PRWDWUWSWEWCDGLVCMOS_H@_UT_Nom_1p8_comment
lvcmos1_utnom_3p3_h PRWDWUWSWEWCDGLVCMOS_H@_UT_Nom_3p3_comment
lvcmos1_utslow_1p8_h PRWDWUWSWEWCDGLVCMOS_H@_UT_Slow_1p8_comment
lvcmos1_utslow_3p3_h PRWDWUWSWEWCDGLVCMOS_H@_UT_Slow_3p3_comment
lvcmos1_utfast_1p8_h PRWDWUWSWEWCDGLVCMOS_H@_UT_Fast_1p8_comment
lvcmos1_utfast_3p3_h PRWDWUWSWEWCDGLVCMOS_H@_UT_Fast_3p3_comment
[Model Selector] LVCMOS_V
lvcmos0_nom_1p8_v PRWDWUWSWEWCDGLVCMOS_V@_Nom_1p8_comment
lvcmos0_nom_3p3_v PRWDWUWSWEWCDGLVCMOS_V@_Nom_3p3_comment
lvcmos0_slow_1p8_v PRWDWUWSWEWCDGLVCMOS_V@_Slow_1p8_comment
lvcmos0_slow_3p3_v PRWDWUWSWEWCDGLVCMOS_V@_Slow_3p3_comment
lvcmos0_fast_1p8_v PRWDWUWSWEWCDGLVCMOS_V@_Fast_1p8_comment
lvcmos0_fast_3p3_v PRWDWUWSWEWCDGLVCMOS_V@_Fast_3p3_comment
lvcmos0_utnom_1p8_v PRWDWUWSWEWCDGLVCMOS_V@_UT_Nom_1p8_comment
lvcmos0_utnom_3p3_v PRWDWUWSWEWCDGLVCMOS_V@_UT_Nom_3p3_comment
lvcmos0_utslow_1p8_v PRWDWUWSWEWCDGLVCMOS_V@_UT_Slow_1p8_comment
lvcmos0_utslow_3p3_v PRWDWUWSWEWCDGLVCMOS_V@_UT_Slow_3p3_comment
lvcmos0_utfast_1p8_v PRWDWUWSWEWCDGLVCMOS_V@_UT_Fast_1p8_comment
lvcmos0_utfast_3p3_v PRWDWUWSWEWCDGLVCMOS_V@_UT_Fast_3p3_comment
|******************* LVDS **********************************
[Model Selector] LVDS
lvds_rx_01   LVDS RX Receiver Permumentation 01
lvds_rx_02   LVDS RX Receiver Permumentation 02
lvds_tx_01   LVDS TX Driver Permumentation 01
lvds_tx_02   LVDS TX Driver Permumentation 02
lvds_tx_03   LVDS TX Driver Permumentation 03
lvds_tx_04   LVDS TX Driver Permumentation 04
lvds_tx_05   LVDS TX Driver Permumentation 05
lvds_tx_06   LVDS TX Driver Permumentation 06
lvds_tx_07   LVDS TX Driver Permumentation 07
lvds_tx_08   LVDS TX Driver Permumentation 08
lvds_tx_09   LVDS TX Driver Permumentation 09
lvds_tx_10   LVDS TX Driver Permumentation 10
lvds_tx_11   LVDS TX Driver Permumentation 11
lvds_tx_12   LVDS TX Driver Permumentation 12
lvds_tx_13   LVDS TX Driver Permumentation 13
lvds_tx_14   LVDS TX Driver Permumentation 14
lvds_tx_15   LVDS TX Driver Permumentation 15
lvds_tx_16   LVDS TX Driver Permumentation 16
lvds_tx_17   LVDS TX Driver Permumentation 17
lvds_tx_18   LVDS TX Driver Permumentation 18
lvds_tx_19   LVDS TX Driver Permumentation 19
lvds_tx_20   LVDS TX Driver Permumentation 20
lvds_tx_21   LVDS TX Driver Permumentation 21
lvds_tx_22   LVDS TX Driver Permumentation 22
lvds_tx_23   LVDS TX Driver Permumentation 23
lvds_tx_24   LVDS TX Driver Permumentation 24
[Model Selector] IIC_H
Cell18_0_0 PRBOPDDGZIIC_H@HSMODE_HSMCSE=0_0_comment 1.8V
Cell18_0_1 PRBOPDDGZIIC_H@HSMODE_HSMCSE=0_1_comment 1.8V
Cell18_0_2 PRBOPDDGZIIC_H@HSMODE_HSMCSE=1_0_comment 1.8V
Cell18_0_3 PRBOPDDGZIIC_H@HSMODE_HSMCSE=1_1_comment 1.8V
Cell33_0_0 PRBOPDDGZIIC_H@HSMODE_HSMCSE=0_0_comment
Cell33_0_1 PRBOPDDGZIIC_H@HSMODE_HSMCSE=0_1_comment
Cell33_0_2 PRBOPDDGZIIC_H@HSMODE_HSMCSE=1_0_comment
Cell33_0_3 PRBOPDDGZIIC_H@HSMODE_HSMCSE=1_1_comment
|***************** RESET ************************************************
[Model Selector] RESET_H
reset18_0_0 PDIDGZRESET_H
|   EMMC
[MODEL SELECTOR] EMMC
emmc51_io_tx33ohm   33ohm DRIVER
emmc51_io_tx40ohm   40ohm DRIVER
emmc51_io_tx50ohm   50ohm DRIVER
emmc51_io_tx66ohm   66ohm DRIVER
emmc51_io_tx100ohm  100ohm DRIVER
emmc51_io_txod   Open drain DRIVER
|******************** Package Model *************************************
[Define Package Model]   ibis_j7es_sck_181218
[Manufacturer]   TI
[OEM]   TI
[Description]   FCBGA
|[Number of Sections]   1
[Number of Pins]   551
[Pin Numbers]
|[Pin Name]  Net Number   Net Name   Net's All Pins
U7	|	1	CAP_VDDS0	U7
K23	|	2	CAP_VDDS0_MCU	K23
AB21	|	3	CAP_VDDS1	AB21
J18	|	4	CAP_VDDS1_MCU	J18
Y18	|	5	CAP_VDDS2	Y18
J19	|	6	CAP_VDDS2_MCU	J19
W21	|	7	CAP_VDDS3	W21
AA22	|	8	CAP_VDDS4	AA22
R22	|	9	CAP_VDDS5	R22
V22	|	10	CAP_VDDS6	V22
L14	|	11	VDDAR_CORE	L14
	|			V13
	|			V16
	|			W19
L11	|	12	VDDAR_CPU	L11
	|			W12
K19	|	13	VDDAR_MCU	K19
	|			T19
H17	|	14	VDDA_0P8_CSIRX	H17
G12	|	15	VDDA_0P8_DP	G12
	|			J12
G14	|	16	VDDA_0P8_DP_C	G14
	|			H13
H15	|	17	VDDA_0P8_DSITX	H15
J16	|	18	VDDA_0P8_DSITX_C	J16
AA15	|	19	VDDA_0P8_SERDES0_1	AA15
	|			Y14
	|			Y16
AA12	|	20	VDDA_0P8_SERDES2_3	AA12
	|			Y11
	|			Y13
AB14	|	21	VDDA_0P8_SERDES_C0_1	AB14
	|			AB15
AB12	|	22	VDDA_0P8_SERDES_C2_3	AB12
	|			AB13
AB9	|	23	VDDA_0P8_UFS	AB9
AA10	|	24	VDDA_0P8_USB	AA10
G16	|	25	VDDA_1P8_CSIRX	G16
H11	|	26	VDDA_1P8_DP	H11
J14	|	27	VDDA_1P8_DSITX	J14
AC14	|	28	VDDA_1P8_SERDES0_1	AC14
	|			AC15
AC11	|	29	VDDA_1P8_SERDES2_3	AC11
	|			AC12
AC8	|	30	VDDA_1P8_UFS	AC8
AC9	|	31	VDDA_1P8_USB	AC9
AB10	|	32	VDDA_3P3_USB	AB10
N22	|	33	VDDA_ADC0	N22
M23	|	34	VDDA_ADC1	M23
N9	|	35	VDDA_DDR_PLL	N9
G18	|	36	VDDA_MCU_PLLGRP0	G18
P21	|	37	VDDA_MCU_TEMP	P21
W7	|	38	VDDA_MLB	W7
Y20	|	39	VDDA_PLLGRP0	Y20
W17	|	40	VDDA_PLLGRP1	W17
M17	|	41	VDDA_PLLGRP2	M17
L12	|	42	VDDA_PLLGRP3	L12
R11	|	43	VDDA_PLLGRP4	R11
P9	|	44	VDDA_PLLGRP5	P9
W18	|	45	VDDA_PLLGRP6	W18
W8	|	46	VDDA_PLLGRP7	W8
P22	|	47	VDDA_POR_WKUP	P22
W15	|	48	VDDA_TEMP0_1	W15
H9	|	49	VDDA_TEMP2_3	H9
M26	|	50	VDDA_VSYS_MON	M26
H22	|	51	VDDA_WKUP	H22
U8	|	52	VDDSHV0	U8
	|			V7
L22	|	53	VDDSHV0_MCU	L22
	|			M22
AA19	|	54	VDDSHV1	AA19
	|			AA20
	|			AC19
	|			AC20
H19	|	55	VDDSHV1_MCU	H19
	|			H21
	|			J20
AA17	|	56	VDDSHV2	AA17
	|			AB16
	|			AB18
	|			AC17
J22	|	57	VDDSHV2_MCU	J22
	|			K21
V21	|	58	VDDSHV3	V21
	|			W22
AA21	|	59	VDDSHV4	AA21
	|			Y22
T20	|	60	VDDSHV5	T20
	|			T22
U20	|	61	VDDSHV6	U20
	|			U22
A1	|	62	VDDS_DDR	A1
	|			G8
	|			J8
	|			K7
	|			L8
	|			M7
	|			N8
	|			P7
	|			R8
	|			T1
H7	|	63	VDDS_DDR_BIAS	H7
	|			J6
	|			R6
	|			T7
M9	|	64	VDDS_DDR_C	M9
AA8	|	65	VDDS_MMC0	AA8
	|			AB7
	|			Y7
R21	|	66	VDDS_OSC1	R21
J10	|	67	VDD_CORE	J10
	|			K9
	|			K11
	|			K13
	|			K15
	|			K17
	|			L10
	|			L16
	|			L18
	|			M15
	|			N14
	|			N16
	|			N18
	|			P13
	|			P15
	|			P17
	|			R14
	|			R16
	|			R18
	|			R20
	|			T9
	|			T15
	|			T17
	|			U14
	|			U16
	|			U18
	|			V15
	|			V17
	|			V20
	|			W14
N10	|	68	VDD_CPU	N10
	|			P11
	|			R10
	|			R12
	|			U10
	|			V9
	|			V11
	|			W10
Y9	|	69	VDD_DLL_MMC0	Y9
L20	|	70	VDD_MCU	L20
	|			M19
	|			M21
	|			N20
	|			P19
V19	|	71	VDD_VMON_EXT_MON	V19
AJ29	|	72	ATEST0	AJ29
E18	|	73	CSI0_ATB_0_H	E18
F18	|	74	CSI0_ATB_1_H	F18
B20	|	75	CSI0_RXCLKN	B20
A21	|	76	CSI0_RXCLKP	A21
B19	|	77	CSI0_RXN0	B19
D18	|	78	CSI0_RXN1	D18
D17	|	79	CSI0_RXN2	D17
E16	|	80	CSI0_RXN3	E16
A20	|	81	CSI0_RXP0	A20
C19	|	82	CSI0_RXP1	C19
C18	|	83	CSI0_RXP2	C18
E17	|	84	CSI0_RXP3	E17
F16	|	85	CSI0_RXRCALIB	F16
G10	|	86	CSI1_ATB_0_H	G10
F11	|	87	CSI1_ATB_1_H	F11
B17	|	88	CSI1_RXCLKN	B17
A18	|	89	CSI1_RXCLKP	A18
B16	|	90	CSI1_RXN0	B16
D15	|	91	CSI1_RXN1	D15
D14	|	92	CSI1_RXN2	D14
E13	|	93	CSI1_RXN3	E13
A17	|	94	CSI1_RXP0	A17
C16	|	95	CSI1_RXP1	C16
C15	|	96	CSI1_RXP2	C15
E14	|	97	CSI1_RXP3	E14
F15	|	98	CSI1_RXRCALIB	F15
N6	|	99	DDR0_ATB0	N6
L6	|	100	DDR0_ATB1	L6
G4	|	101	DDR0_CA0	G4
H3	|	102	DDR0_CA1	H3
K5	|	103	DDR0_CA2	K5
J4	|	104	DDR0_CA3	J4
K2	|	105	DDR0_CA4	K2
H5	|	106	DDR0_CA5	H5
H2	|	107	DDR0_CAL0	H2
G3	|	108	DDR0_CKE0	G3
J3	|	109	DDR0_CKE1	J3
J1	|	110	DDR0_CKN	J1
H1	|	111	DDR0_CKP	H1
J5	|	112	DDR0_CSN0_0	J5
K3	|	113	DDR0_CSN0_1	K3
G5	|	114	DDR0_CSN1_0	G5
J2	|	115	DDR0_CSN1_1	J2
A3	|	116	DDR0_DM0	A3
E4	|	117	DDR0_DM1	E4
N1	|	118	DDR0_DM2	N1
R5	|	119	DDR0_DM3	R5
A5	|	120	DDR0_DQ0	A5
A6	|	121	DDR0_DQ1	A6
B5	|	122	DDR0_DQ2	B5
C2	|	123	DDR0_DQ3	C2
B4	|	124	DDR0_DQ4	B4
C3	|	125	DDR0_DQ5	C3
A2	|	126	DDR0_DQ6	A2
A4	|	127	DDR0_DQ7	A4
D1	|	128	DDR0_DQ8	D1
C4	|	129	DDR0_DQ9	C4
F1	|	130	DDR0_DQ10	F1
G2	|	131	DDR0_DQ11	G2
F2	|	132	DDR0_DQ12	F2
F3	|	133	DDR0_DQ13	F3
D3	|	134	DDR0_DQ14	D3
F5	|	135	DDR0_DQ15	F5
L5	|	136	DDR0_DQ16	L5
M5	|	137	DDR0_DQ17	M5
N5	|	138	DDR0_DQ18	N5
L4	|	139	DDR0_DQ19	L4
L2	|	140	DDR0_DQ20	L2
L1	|	141	DDR0_DQ21	L1
N2	|	142	DDR0_DQ22	N2
N4	|	143	DDR0_DQ23	N4
T3	|	144	DDR0_DQ24	T3
T2	|	145	DDR0_DQ25	T2
P2	|	146	DDR0_DQ26	P2
P3	|	147	DDR0_DQ27	P3
P5	|	148	DDR0_DQ28	P5
R4	|	149	DDR0_DQ29	R4
T4	|	150	DDR0_DQ30	T4
T5	|	151	DDR0_DQ31	T5
B1	|	152	DDR0_DQS0N	B1
B2	|	153	DDR0_DQS0P	B2
E2	|	154	DDR0_DQS1N	E2
E3	|	155	DDR0_DQS1P	E3
M2	|	156	DDR0_DQS2N	M2
M3	|	157	DDR0_DQS2P	M3
R1	|	158	DDR0_DQS3N	R1
R2	|	159	DDR0_DQS3P	R2
K6	|	160	DDR0_RESETN	K6
P6	|	161	DDR_RET	P6
G6	|	162	DP0_AUXN	G6
F7	|	163	DP0_AUXP	F7
F6	|	164	DP0_AUX_ATB_0	F6
E6	|	165	DP0_AUX_ATB_1	E6
G9	|	166	DSI_ATB_0_H	G9
F10	|	167	DSI_ATB_1_H	F10
E10	|	168	DSI_TXCLKN	E10
E11	|	169	DSI_TXCLKP	E11
D11	|	170	DSI_TXN0	D11
D12	|	171	DSI_TXN1	D12
B13	|	172	DSI_TXN2	B13
B14	|	173	DSI_TXN3	B14
C12	|	174	DSI_TXP0	C12
C13	|	175	DSI_TXP1	C13
A14	|	176	DSI_TXP2	A14
A15	|	177	DSI_TXP3	A15
F12	|	178	DSI_TXRCALIB	F12
U2	|	179	ECAP0_IN_APWM_OUT	U2
C26	|	180	EMU0	C26
B29	|	181	EMU1	B29
AC18	|	182	EXTINTN	AC18
U3	|	183	EXT_REFCLK1	U3
AC5	|	184	I2C0_SCL	AC5
AA5	|	185	I2C0_SDA	AA5
Y6	|	186	I2C1_SCL	Y6
AA6	|	187	I2C1_SDA	AA6
W2	|	188	I3C0_SCL	W2
W1	|	189	I3C0_SDA	W1
P26	|	190	IFORCE	P26
N25	|	191	MAIN_ATEST	N25
W5	|	192	MCAN0_RX	W5
W6	|	193	MCAN0_TX	W6
W3	|	194	MCAN1_RX	W3
V4	|	195	MCAN1_TX	V4
K25	|	196	MCU_ADC0_AIN0	K25
K26	|	197	MCU_ADC0_AIN1	K26
K28	|	198	MCU_ADC0_AIN2	K28
L28	|	199	MCU_ADC0_AIN3	L28
K24	|	200	MCU_ADC0_AIN4	K24
K27	|	201	MCU_ADC0_AIN5	K27
K29	|	202	MCU_ADC0_AIN6	K29
L29	|	203	MCU_ADC0_AIN7	L29
N23	|	204	MCU_ADC1_AIN0	N23
M25	|	205	MCU_ADC1_AIN1	M25
L24	|	206	MCU_ADC1_AIN2	L24
L26	|	207	MCU_ADC1_AIN3	L26
N24	|	208	MCU_ADC1_AIN4	N24
M24	|	209	MCU_ADC1_AIN5	M24
L25	|	210	MCU_ADC1_AIN6	L25
L27	|	211	MCU_ADC1_AIN7	L27
J26	|	212	MCU_I2C0_SCL	J26
H25	|	213	MCU_I2C0_SDA	H25
D26	|	214	MCU_I3C0_SCL	D26
D25	|	215	MCU_I3C0_SDA	D25
C29	|	216	MCU_MCAN0_RX	C29
D29	|	217	MCU_MCAN0_TX	D29
F23	|	218	MCU_MDIO0_MDC	F23
E23	|	219	MCU_MDIO0_MDIO	E23
E20	|	220	MCU_OSPI0_CLK	E20
F19	|	221	MCU_OSPI0_CSN0	F19
E19	|	222	MCU_OSPI0_CSN1	E19
D20	|	223	MCU_OSPI0_D0	D20
G19	|	224	MCU_OSPI0_D1	G19
G20	|	225	MCU_OSPI0_D2	G20
F20	|	226	MCU_OSPI0_D3	F20
F21	|	227	MCU_OSPI0_D4	F21
E21	|	228	MCU_OSPI0_D5	E21
B22	|	229	MCU_OSPI0_D6	B22
G21	|	230	MCU_OSPI0_D7	G21
D21	|	231	MCU_OSPI0_DQS	D21
C21	|	232	MCU_OSPI0_LBCLKO	C21
F22	|	233	MCU_OSPI1_CLK	F22
C22	|	234	MCU_OSPI1_CSN0	C22
E22	|	235	MCU_OSPI1_CSN1	E22
D22	|	236	MCU_OSPI1_D0	D22
G22	|	237	MCU_OSPI1_D1	G22
D23	|	238	MCU_OSPI1_D2	D23
C23	|	239	MCU_OSPI1_D3	C23
B23	|	240	MCU_OSPI1_DQS	B23
A23	|	241	MCU_OSPI1_LBCLKO	A23
H23	|	242	MCU_PORZ	H23
B28	|	243	MCU_PORZ_OUT	B28
C27	|	244	MCU_RESETSTATZ	C27
D28	|	245	MCU_RESETZ	D28
B24	|	246	MCU_RGMII1_RD0	B24
A24	|	247	MCU_RGMII1_RD1	A24
D24	|	248	MCU_RGMII1_RD2	D24
A25	|	249	MCU_RGMII1_RD3	A25
C24	|	250	MCU_RGMII1_RXC	C24
C25	|	251	MCU_RGMII1_RX_CTL	C25
B25	|	252	MCU_RGMII1_TD0	B25
A26	|	253	MCU_RGMII1_TD1	A26
A27	|	254	MCU_RGMII1_TD2	A27
A28	|	255	MCU_RGMII1_TD3	A28
B26	|	256	MCU_RGMII1_TXC	B26
B27	|	257	MCU_RGMII1_TX_CTL	B27
D27	|	258	MCU_SAFETY_ERRORN	D27
E27	|	259	MCU_SPI0_CLK	E27
E25	|	260	MCU_SPI0_CS0	E25
E24	|	261	MCU_SPI0_D0	E24
E28	|	262	MCU_SPI0_D1	E28
V24	|	263	MDIO0_MDC	V24
V26	|	264	MDIO0_MDIO	V26
AE2	|	265	MLB0_MLBCN	AE2
AD2	|	266	MLB0_MLBCP	AD2
AD3	|	267	MLB0_MLBDN	AD3
AC3	|	268	MLB0_MLBDP	AC3
AC1	|	269	MLB0_MLBSN	AC1
AD1	|	270	MLB0_MLBSP	AD1
AE1	|	271	MMC0_CALPAD	AE1
AF1	|	272	MMC0_CLK	AF1
AE3	|	273	MMC0_CMD	AE3
AG2	|	274	MMC0_DAT0	AG2
AH1	|	275	MMC0_DAT1	AH1
AG3	|	276	MMC0_DAT2	AG3
AF4	|	277	MMC0_DAT3	AF4
AE5	|	278	MMC0_DAT4	AE5
AF3	|	279	MMC0_DAT5	AF3
AG1	|	280	MMC0_DAT6	AG1
AF2	|	281	MMC0_DAT7	AF2
AE4	|	282	MMC0_DS	AE4
AD4	|	283	MMC0_VCTRL_TP	AD4
P25	|	284	MMC1_CLK	P25
R29	|	285	MMC1_CMD	R29
R24	|	286	MMC1_DAT0	R24
P24	|	287	MMC1_DAT1	P24
R25	|	288	MMC1_DAT2	R25
R26	|	289	MMC1_DAT3	R26
P23	|	290	MMC1_SDCD	P23
R28	|	291	MMC1_SDWP	R28
T26	|	292	MMC2_CLK	T26
T25	|	293	MMC2_CMD	T25
T24	|	294	MMC2_DAT0	T24
T27	|	295	MMC2_DAT1	T27
T29	|	296	MMC2_DAT2	T29
T28	|	297	MMC2_DAT3	T28
P29	|	298	OSC1_XI	P29
P27	|	299	OSC1_XO	P27
AE17	|	300	PCIE_REFCLK0N	AE17
AD16	|	301	PCIE_REFCLK0P	AD16
AE14	|	302	PCIE_REFCLK1N	AE14
AD15	|	303	PCIE_REFCLK1P	AD15
AE11	|	304	PCIE_REFCLK2N	AE11
AD12	|	305	PCIE_REFCLK2P	AD12
AE9	|	306	PCIE_REFCLK3N	AE9
AD10	|	307	PCIE_REFCLK3P	AD10
E26	|	308	PMIC_POWER_EN0	E26
G23	|	309	PMIC_POWER_EN1	G23
J24	|	310	PORZ	J24
U1	|	311	PORZ_OUT	U1
AA27	|	312	PRG0_MDIO0_MDC	AA27
Y26	|	313	PRG0_MDIO0_MDIO	Y26
AF28	|	314	PRG0_PRU0_GPO0	AF28
AE28	|	315	PRG0_PRU0_GPO1	AE28
AE27	|	316	PRG0_PRU0_GPO2	AE27
AD26	|	317	PRG0_PRU0_GPO3	AD26
AD25	|	318	PRG0_PRU0_GPO4	AD25
AC29	|	319	PRG0_PRU0_GPO5	AC29
AE26	|	320	PRG0_PRU0_GPO6	AE26
AC28	|	321	PRG0_PRU0_GPO7	AC28
AC27	|	322	PRG0_PRU0_GPO8	AC27
AB26	|	323	PRG0_PRU0_GPO9	AB26
AB25	|	324	PRG0_PRU0_GPO10	AB25
AJ28	|	325	PRG0_PRU0_GPO11	AJ28
AH27	|	326	PRG0_PRU0_GPO12	AH27
AH29	|	327	PRG0_PRU0_GPO13	AH29
AG28	|	328	PRG0_PRU0_GPO14	AG28
AG27	|	329	PRG0_PRU0_GPO15	AG27
AH28	|	330	PRG0_PRU0_GPO16	AH28
AB24	|	331	PRG0_PRU0_GPO17	AB24
AB29	|	332	PRG0_PRU0_GPO18	AB29
AB28	|	333	PRG0_PRU0_GPO19	AB28
AE29	|	334	PRG0_PRU1_GPO0	AE29
AD28	|	335	PRG0_PRU1_GPO1	AD28
AD27	|	336	PRG0_PRU1_GPO2	AD27
AC25	|	337	PRG0_PRU1_GPO3	AC25
AD29	|	338	PRG0_PRU1_GPO4	AD29
AB27	|	339	PRG0_PRU1_GPO5	AB27
AC26	|	340	PRG0_PRU1_GPO6	AC26
AA24	|	341	PRG0_PRU1_GPO7	AA24
AA28	|	342	PRG0_PRU1_GPO8	AA28
Y24	|	343	PRG0_PRU1_GPO9	Y24
AA25	|	344	PRG0_PRU1_GPO10	AA25
AG26	|	345	PRG0_PRU1_GPO11	AG26
AF27	|	346	PRG0_PRU1_GPO12	AF27
AF26	|	347	PRG0_PRU1_GPO13	AF26
AE25	|	348	PRG0_PRU1_GPO14	AE25
AF29	|	349	PRG0_PRU1_GPO15	AF29
AG29	|	350	PRG0_PRU1_GPO16	AG29
Y25	|	351	PRG0_PRU1_GPO17	Y25
AA26	|	352	PRG0_PRU1_GPO18	AA26
AA29	|	353	PRG0_PRU1_GPO19	AA29
AD18	|	354	PRG1_MDIO0_MDC	AD18
AD19	|	355	PRG1_MDIO0_MDIO	AD19
AC23	|	356	PRG1_PRU0_GPO0	AC23
AG22	|	357	PRG1_PRU0_GPO1	AG22
AF22	|	358	PRG1_PRU0_GPO2	AF22
AJ23	|	359	PRG1_PRU0_GPO3	AJ23
AH23	|	360	PRG1_PRU0_GPO4	AH23
AD20	|	361	PRG1_PRU0_GPO5	AD20
AD22	|	362	PRG1_PRU0_GPO6	AD22
AE20	|	363	PRG1_PRU0_GPO7	AE20
AJ20	|	364	PRG1_PRU0_GPO8	AJ20
AG20	|	365	PRG1_PRU0_GPO9	AG20
AD21	|	366	PRG1_PRU0_GPO10	AD21
AF24	|	367	PRG1_PRU0_GPO11	AF24
AJ24	|	368	PRG1_PRU0_GPO12	AJ24
AG24	|	369	PRG1_PRU0_GPO13	AG24
AD24	|	370	PRG1_PRU0_GPO14	AD24
AC24	|	371	PRG1_PRU0_GPO15	AC24
AE24	|	372	PRG1_PRU0_GPO16	AE24
AJ21	|	373	PRG1_PRU0_GPO17	AJ21
AE21	|	374	PRG1_PRU0_GPO18	AE21
AH21	|	375	PRG1_PRU0_GPO19	AH21
AE22	|	376	PRG1_PRU1_GPO0	AE22
AG23	|	377	PRG1_PRU1_GPO1	AG23
AF23	|	378	PRG1_PRU1_GPO2	AF23
AD23	|	379	PRG1_PRU1_GPO3	AD23
AH24	|	380	PRG1_PRU1_GPO4	AH24
AG21	|	381	PRG1_PRU1_GPO5	AG21
AE23	|	382	PRG1_PRU1_GPO6	AE23
AC21	|	383	PRG1_PRU1_GPO7	AC21
Y23	|	384	PRG1_PRU1_GPO8	Y23
AF21	|	385	PRG1_PRU1_GPO9	AF21
AB23	|	386	PRG1_PRU1_GPO10	AB23
AJ25	|	387	PRG1_PRU1_GPO11	AJ25
AH25	|	388	PRG1_PRU1_GPO12	AH25
AG25	|	389	PRG1_PRU1_GPO13	AG25
AH26	|	390	PRG1_PRU1_GPO14	AH26
AJ27	|	391	PRG1_PRU1_GPO15	AJ27
AJ26	|	392	PRG1_PRU1_GPO16	AJ26
AC22	|	393	PRG1_PRU1_GPO17	AC22
AJ22	|	394	PRG1_PRU1_GPO18	AJ22
AH22	|	395	PRG1_PRU1_GPO19	AH22
T6	|	396	RESETSTATZ	T6
C28	|	397	RESET_REQZ	C28
T23	|	398	RGMII5_RD0	T23
R23	|	399	RGMII5_RD1	R23
U24	|	400	RGMII5_RD2	U24
U27	|	401	RGMII5_RD3	U27
U25	|	402	RGMII5_RXC	U25
U26	|	403	RGMII5_RX_CTL	U26
U28	|	404	RGMII5_TD0	U28
V27	|	405	RGMII5_TD1	V27
V29	|	406	RGMII5_TD2	V29
V28	|	407	RGMII5_TD3	V28
U29	|	408	RGMII5_TXC	U29
U23	|	409	RGMII5_TX_CTL	U23
W25	|	410	RGMII6_RD0	W25
W24	|	411	RGMII6_RD1	W24
Y27	|	412	RGMII6_RD2	Y27
Y29	|	413	RGMII6_RD3	Y29
W26	|	414	RGMII6_RXC	W26
V23	|	415	RGMII6_RX_CTL	V23
W27	|	416	RGMII6_TD0	W27
V25	|	417	RGMII6_TD1	V25
W28	|	418	RGMII6_TD2	W28
W23	|	419	RGMII6_TD3	W23
W29	|	420	RGMII6_TXC	W29
Y28	|	421	RGMII6_TX_CTL	Y28
AE18	|	422	SERDES0_REXT	AE18
AH19	|	423	SERDES0_RX0_N	AH19
AJ18	|	424	SERDES0_RX0_P	AJ18
AH18	|	425	SERDES0_RX1_N	AH18
AJ17	|	426	SERDES0_RX1_P	AJ17
AF19	|	427	SERDES0_TX0_N	AF19
AG18	|	428	SERDES0_TX0_P	AG18
AF18	|	429	SERDES0_TX1_N	AF18
AG17	|	430	SERDES0_TX1_P	AG17
AE13	|	431	SERDES1_REXT	AE13
AH15	|	432	SERDES1_RX0_N	AH15
AJ14	|	433	SERDES1_RX0_P	AJ14
AH16	|	434	SERDES1_RX1_N	AH16
AJ15	|	435	SERDES1_RX1_P	AJ15
AF15	|	436	SERDES1_TX0_N	AF15
AG14	|	437	SERDES1_TX0_P	AG14
AF16	|	438	SERDES1_TX1_N	AF16
AG15	|	439	SERDES1_TX1_P	AG15
AD13	|	440	SERDES2_REXT	AD13
AH13	|	441	SERDES2_RX0_N	AH13
AJ12	|	442	SERDES2_RX0_P	AJ12
AH12	|	443	SERDES2_RX1_N	AH12
AJ11	|	444	SERDES2_RX1_P	AJ11
AF13	|	445	SERDES2_TX0_N	AF13
AG12	|	446	SERDES2_TX0_P	AG12
AF12	|	447	SERDES2_TX1_N	AF12
AG11	|	448	SERDES2_TX1_P	AG11
AE8	|	449	SERDES3_REXT	AE8
AH9	|	450	SERDES3_RX0_N	AH9
AJ8	|	451	SERDES3_RX0_P	AJ8
AH10	|	452	SERDES3_RX1_N	AH10
AJ9	|	453	SERDES3_RX1_P	AJ9
AF9	|	454	SERDES3_TX0_N	AF9
AG8	|	455	SERDES3_TX0_P	AG8
AF10	|	456	SERDES3_TX1_N	AF10
AG9	|	457	SERDES3_TX1_P	AG9
E7	|	458	SERDES4_REFCLK_N	E7
E8	|	459	SERDES4_REFCLK_P	E8
F9	|	460	SERDES4_REXT	F9
D9	|	461	SERDES4_RX0_N	D9
C10	|	462	SERDES4_RX0_P	C10
D8	|	463	SERDES4_RX1_N	D8
C9	|	464	SERDES4_RX1_P	C9
D6	|	465	SERDES4_RX2_N	D6
C7	|	466	SERDES4_RX2_P	C7
D5	|	467	SERDES4_RX3_N	D5
C6	|	468	SERDES4_RX3_P	C6
B11	|	469	SERDES4_TX0_N	B11
A12	|	470	SERDES4_TX0_P	A12
B10	|	471	SERDES4_TX1_N	B10
A11	|	472	SERDES4_TX1_P	A11
B8	|	473	SERDES4_TX2_N	B8
A9	|	474	SERDES4_TX2_P	A9
B7	|	475	SERDES4_TX3_N	B7
A8	|	476	SERDES4_TX3_P	A8
U4	|	477	SOC_SAFETY_ERRORN	U4
AA1	|	478	SPI0_CLK	AA1
AA2	|	479	SPI0_CS0	AA2
Y4	|	480	SPI0_CS1	Y4
AB5	|	481	SPI0_D0	AB5
AA3	|	482	SPI0_D1	AA3
Y1	|	483	SPI1_CLK	Y1
Y3	|	484	SPI1_CS0	Y3
W4	|	485	SPI1_CS1	W4
Y5	|	486	SPI1_D0	Y5
Y2	|	487	SPI1_D1	Y2
E29	|	488	TCK	E29
V1	|	489	TDI	V1
V3	|	490	TDO	V3
F13	|	491	TEMP_DIODE_P	F13
V6	|	492	TIMER_IO0	V6
V5	|	493	TIMER_IO1	V5
V2	|	494	TMS	V2
F24	|	495	TRSTN	F24
AC2	|	496	UART0_CTSN	AC2
AB1	|	497	UART0_RTSN	AB1
AB2	|	498	UART0_RXD	AB2
AB3	|	499	UART0_TXD	AB3
AC4	|	500	UART1_CTSN	AC4
AD5	|	501	UART1_RTSN	AD5
AA4	|	502	UART1_RXD	AA4
AB4	|	503	UART1_TXD	AB4
AE6	|	504	UFS0_REF_CLK	AE6
AD6	|	505	UFS0_RSTN	AD6
AH3	|	506	UFS0_RX_DN0	AH3
AH4	|	507	UFS0_RX_DN1	AH4
AJ2	|	508	UFS0_RX_DP0	AJ2
AJ3	|	509	UFS0_RX_DP1	AJ3
AG6	|	510	UFS0_TX_DN0	AG6
AG5	|	511	UFS0_TX_DN1	AG5
AF7	|	512	UFS0_TX_DP0	AF7
AF6	|	513	UFS0_TX_DP1	AF6
AJ5	|	514	USB0_DM	AJ5
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[Model Data]
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[End Model Data]
[End Package Model]
| Models and submodels in the file (143): lvcmos1_nom_1p8_h (I/O), lvcmos0_nom_1p8_v (I/O), lvcmos1_nom_3p3_h (I/O), lvcmos0_nom_3p3_v (I/O), lvcmos1_slow_1p8_h (I/O), lvcmos0_slow_1p8_v (I/O), lvcmos1_slow_3p3_h (I/O), lvcmos0_slow_3p3_v (I/O), lvcmos1_fast_1p8_h (I/O), lvcmos0_fast_1p8_v (I/O), lvcmos1_fast_3p3_h (I/O), lvcmos0_fast_3p3_v (I/O), lvcmos1_utnom_1p8_h (I/O), lvcmos0_utnom_1p8_v (I/O), lvcmos1_utnom_3p3_h (I/O), lvcmos0_utnom_3p3_v (I/O), lvcmos1_utslow_1p8_h (I/O), lvcmos0_utslow_1p8_v (I/O), lvcmos1_utslow_3p3_h (I/O), lvcmos0_utslow_3p3_v (I/O), lvcmos1_utfast_1p8_h (I/O), lvcmos0_utfast_1p8_v (I/O), lvcmos1_utfast_3p3_h (I/O), lvcmos0_utfast_3p3_v (I/O), sdio1_r33_1p8_h (I/O), sdio1_r33_3p3_h (I/O), sdio1_r40_1p8_h (I/O), sdio1_r40_3p3_h (I/O), sdio1_r50_1p8_h (I/O), sdio1_r50_3p3_h (I/O), sdio1_r66_1p8_h (I/O), sdio1_r66_3p3_h (I/O), sdio1_utr33_1p8_h (I/O), sdio1_utr33_3p3_h (I/O), sdio1_utr40_1p8_h (I/O), sdio1_utr40_3p3_h (I/O), sdio1_utr50_1p8_h (I/O), sdio1_utr50_3p3_h (I/O), sdio1_utr66_1p8_h (I/O), sdio1_utr66_3p3_h (I/O), lpddr4_odt_120 (Input), lpddr4_odt_120_diff (Input), lpddr4_ocd_120p_120n (I/O), lpddr4_ocd_240p_240n (I/O), lpddr4_odt_240 (Input), lpddr4_ocd_40p_40n (I/O), lpddr4_odt_40 (Input), lpddr4_ocd_48p_48n (I/O), lpddr4_odt_48 (Input), lpddr4_ocd_60p_60n (I/O), lpddr4_odt_60 (Input), lpddr4_ocd_80p_80n (I/O), lpddr4_odt_80 (Input), lpddr4_odt_off (Input), lpddr4_ocd_120pd_60p_40n (I/O), lpddr4_ocd_120p_120n_diff (I/O), lpddr4_ocd_240p_240n_diff (I/O), lpddr4_odt_240_diff (Input), lpddr4_ocd_40p_40n_diff (I/O), lpddr4_odt_40_diff (Input), lpddr4_ocd_48p_48n_diff (I/O), lpddr4_odt_48_diff (Input), lpddr4_ocd_60p_60n_diff (I/O), lpddr4_odt_60_diff (Input), lpddr4_ocd_80p_80n_diff (I/O), lpddr4_ocd_120pd_60p_40n_diff (I/O), lpddr4_odt_80_diff (Input), lpddr4_odt_off_diff (Input), lpddr4_ocd_120pd_48p_40n (I/O), lpddr4_ocd_120pd_48p_40n_diff (I/O), lp4x_ocd_40p_40n (I/O), lp4x_ocd_120p_120n (I/O), lp4x_ocd_48p_48n (I/O), lp4x_ocd_34p_34n (I/O), lp4x_ocd_80p_80n (I/O), lp4x_ocd_240p_240n (I/O), lp4x_ocd_60p_60n (I/O), lp4x_0p6_ocd_80p_80n (I/O), lp4x_0p6_ocd_40p_40n (I/O), lp4x_odt_120 (Input)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
